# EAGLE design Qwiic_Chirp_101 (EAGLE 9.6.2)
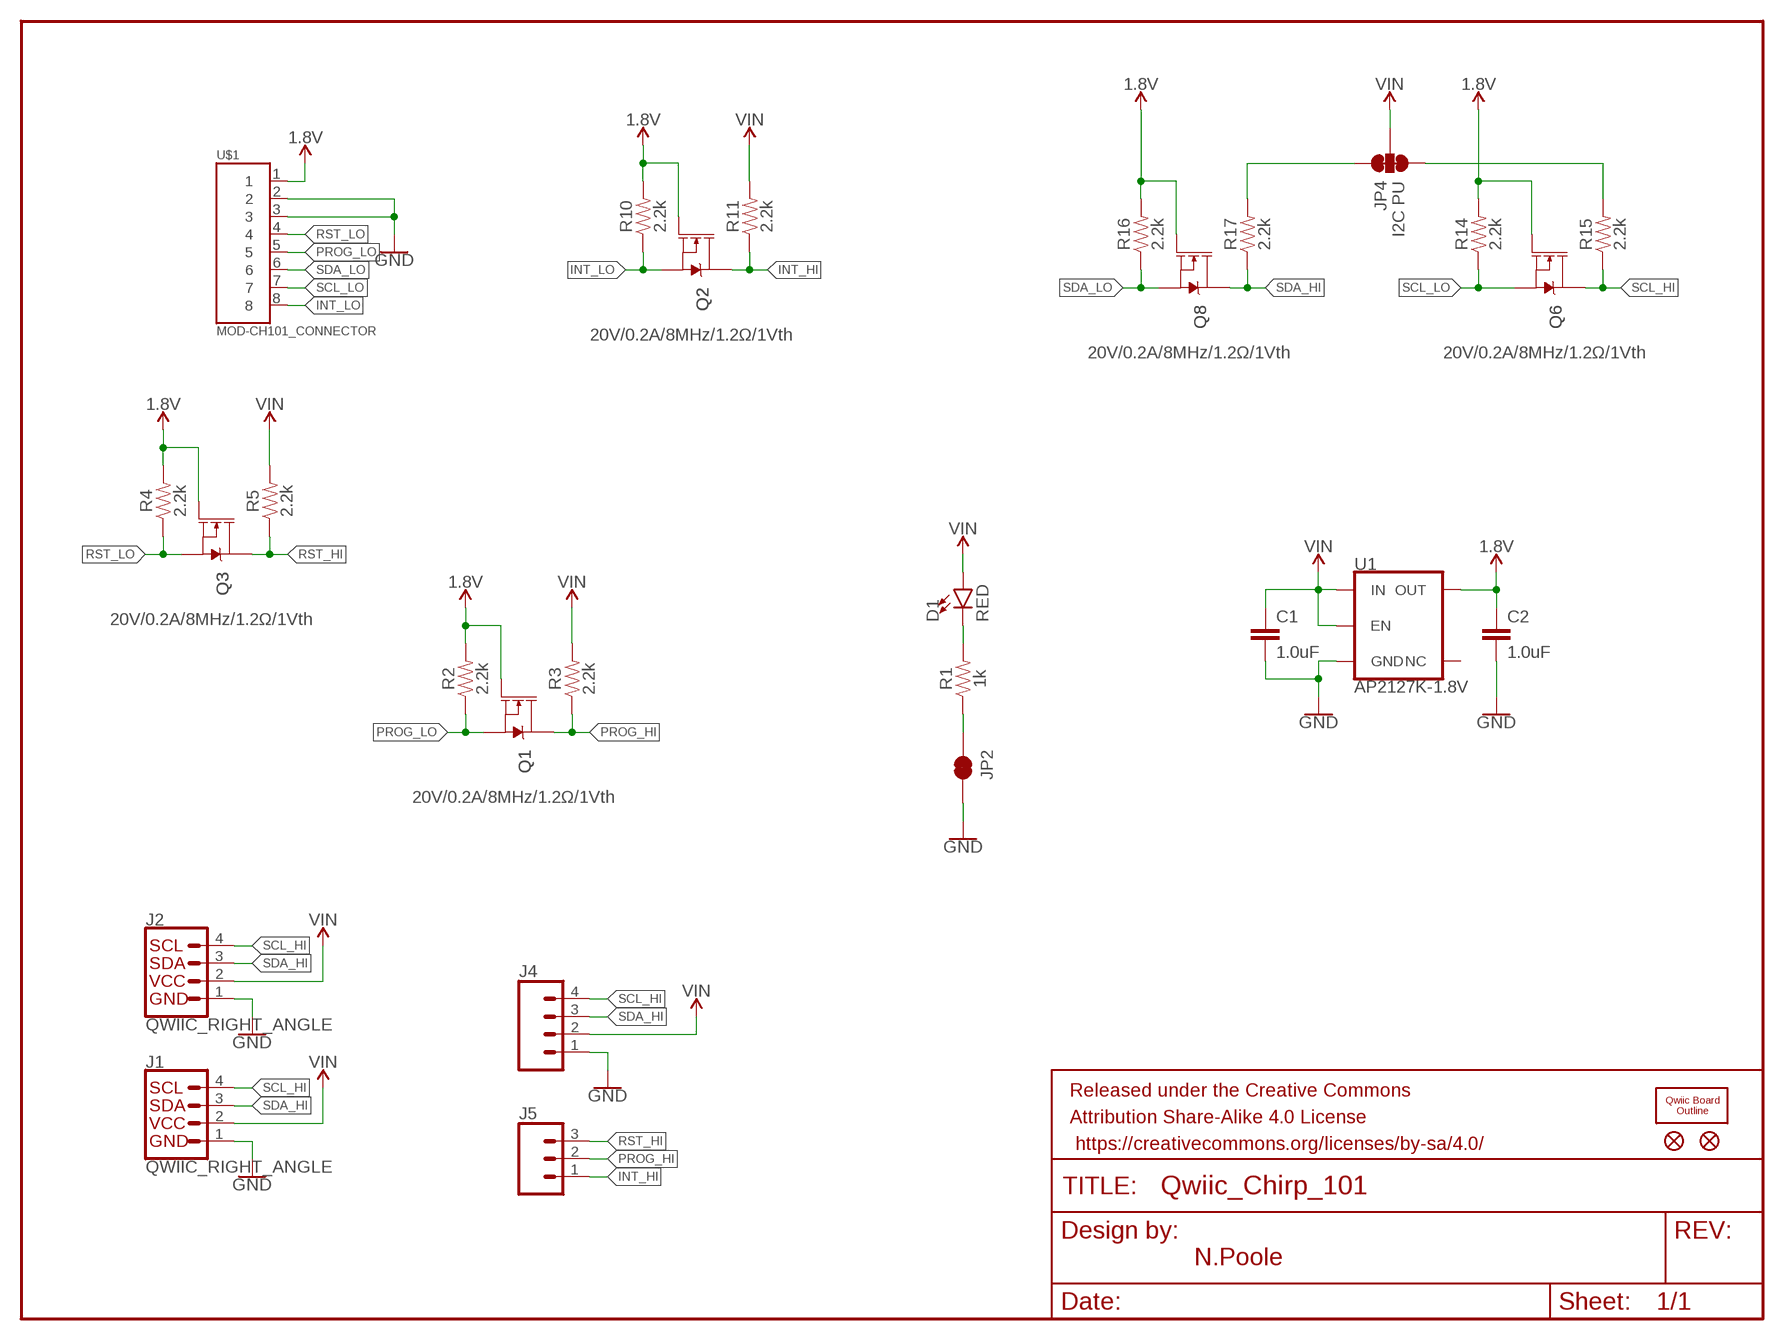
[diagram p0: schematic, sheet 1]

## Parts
C1  1.0uF  1.0UF-0603-16V-10%  [0603]
C2  1.0uF  1.0UF-0603-16V-10%  [0603]
D1  RED  LED-RED0603  [LED-0603]
FD1  FIDUCIALUFIDUCIAL  [FIDUCIAL-MICRO]
FD2  FIDUCIALUFIDUCIAL  [FIDUCIAL-MICRO]
FRAME1  FRAME-LETTERNO_PACKAGE  [DUMMY]
J1  QWIIC_RIGHT_ANGLE  QWIIC_CONNECTORJS-1MM  [JST04_1MM_RA]
J2  QWIIC_RIGHT_ANGLE  QWIIC_CONNECTORJS-1MM  [JST04_1MM_RA]
J4  CONN_041X04_NO_SILK  [1X04_NO_SILK]
J5  CONN_031X03_NO_SILK  [1X03_NO_SILK]
JP2  JUMPER-SMT_2_NC_TRACE_SILK  [SMT-JUMPER_2_NC_TRACE_SILK]
JP4  I2C PU  JUMPER-SMT_3_2-NC_TRACE_SILK  [SMT-JUMPER_3_2-NC_TRACE_SILK]
Q1  20V/0.2A/8MHz/1.2Ω/1Vth  MOSFET-NCH-RE1C002UN  [SOT-416FL]
Q2  20V/0.2A/8MHz/1.2Ω/1Vth  MOSFET-NCH-RE1C002UN  [SOT-416FL]
Q3  20V/0.2A/8MHz/1.2Ω/1Vth  MOSFET-NCH-RE1C002UN  [SOT-416FL]
Q6  20V/0.2A/8MHz/1.2Ω/1Vth  MOSFET-NCH-RE1C002UN  [SOT-416FL]
Q8  20V/0.2A/8MHz/1.2Ω/1Vth  MOSFET-NCH-RE1C002UN  [SOT-416FL]
R1  1k  1KOHM-0603-1/10W-1%  [0603]
R2  2.2k  2.2KOHM-0402T-1/16W-1%  [0402-TIGHT]
R3  2.2k  2.2KOHM-0402T-1/16W-1%  [0402-TIGHT]
R4  2.2k  2.2KOHM-0402T-1/16W-1%  [0402-TIGHT]
R5  2.2k  2.2KOHM-0402T-1/16W-1%  [0402-TIGHT]
R10  2.2k  2.2KOHM-0402T-1/16W-1%  [0402-TIGHT]
R11  2.2k  2.2KOHM-0402T-1/16W-1%  [0402-TIGHT]
R14  2.2k  2.2KOHM-0402T-1/16W-1%  [0402-TIGHT]
R15  2.2k  2.2KOHM-0402T-1/16W-1%  [0402-TIGHT]
R16  2.2k  2.2KOHM-0402T-1/16W-1%  [0402-TIGHT]
R17  2.2k  2.2KOHM-0402T-1/16W-1%  [0402-TIGHT]
U1  AP2127K-1.8V  V_REG_AP2127K-1.8V  [SOT23-5]
U$1  MOD-CH101_CONNECTOR  [FPC_MOLEX5034800800]
U$2  QWIIC_BOARD_OUTLINEH  [QWIIC_BOARD_MOUNT_HOLES]

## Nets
1.8V: C2.1 Q1.1(G) Q2.1(G) Q3.1(G) Q6.1(G) Q8.1(G) R2.2 R4.2 R10.2 R14.2 R16.2 U1.5(OUT) U$1.1
GND: C1.2 C2.2 J1.1 J2.1 J4.1 JP2.2 U1.2(GND) U$1.2 U$1.3
INT_HI: J5.1 Q2.3(D) R11.1
INT_LO: Q2.2(S) R10.1 U$1.8
N$1: D1.C R1.2
N$2: JP4.3 R15.2
N$3: JP4.1 R17.2
N$4: JP2.1 R1.1
PROG_HI: J5.2 Q1.3(D) R3.1
PROG_LO: Q1.2(S) R2.1 U$1.5
RST_HI: J5.3 Q3.3(D) R5.1
RST_LO: Q3.2(S) R4.1 U$1.4
SCL_HI: J1.4 J2.4 J4.4 Q6.3(D) R15.1
SCL_LO: Q6.2(S) R14.1 U$1.7
SDA_HI: J1.3 J2.3 J4.3 Q8.3(D) R17.1
SDA_LO: Q8.2(S) R16.1 U$1.6
VIN: C1.1 D1.A J1.2 J2.2 J4.2 JP4.2 R3.2 R5.2 R11.2 U1.1(IN) U1.3(EN)
Unconnected: U1.4(NC)

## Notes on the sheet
- N.Poole

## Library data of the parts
C1 C2 = SparkFun-Capacitors:1.0UF: 1µF ceramic capacitors; PROD_ID: CAP-00868
D1 = SparkFun-LED:LED-RED: Red SMD LED; PROD_ID: DIO-00819
FD1 FD2 = SparkFun-Aesthetics:FIDUCIAL: Fiducial Alignment Points
FRAME1 = SparkFun-Aesthetics:FRAME-LETTER: Schematic Frame - Letter; DESIGNER: Nobody; VERSION: v01
J1 J2 = SparkFun-Connectors:QWIIC_CONNECTOR: SparkFun I2C Standard Qwiic Connector An SMD 1mm pitch JST connector makes it easy and quick (get it? Qwiic?) to connect I2C devices to each other. The Qwiic system enables fast and solderless connection between popular platforms and various sensors and actuators. We carry 200mm, 100mm, 50mm, and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; PROD_ID: CONN-13694
J4 = SparkFun-Connectors:CONN_04: Multi connection point. Often used as Generic Header-pin footprint for 0.1 inch spaced/style header connections On any of the 0.1 inch spaced packages, you can populate with these: Break Away Headers - Straight (PRT-00116) Break Away Male Headers - Right Angle (PRT-00553) Female Headers (PRT-00115)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; PROD_ID: CONN-09696
J5 = SparkFun-Connectors:CONN_03: Multi connection point. Often used as Generic Header-pin footprint for 0.1 inch spaced/style header connections On any of the 0.1 inch spaced packages, you can populate with these: Break Away Headers - Straight (PRT-00116) Break Away Male Headers - Right Angle (PRT-00553) Female Headers (PRT-00115)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
JP2 = SparkFun-Jumpers:JUMPER-SMT_2_NC_TRACE: Normally closed trace jumper
JP4 = SparkFun-Jumpers:JUMPER-SMT_3_2-NC_TRACE: Normally closed trace jumper (2 of 2 connections) This jumper has a trace between all three pads so they are normally closed (NC). Use a razor knife to open the connection(s). For best results follow the IPC guidelines for cutting traces: Cutout at least 0.063 mm (0.005 in). Remove all loose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
Q1-Q3 Q6 Q8 = SparkFun-DiscreteSemi:MOSFET-NCH: N-channel MOSFETs Voltage controlled devices that allow control of high current outputs. SparkFun Products: SparkFun OpenScale SparkFun Digital Sandbox SparkFun Monster Moto Shield SparkFun MOSFET Power Controller; PROD_ID: TRANS_14399
R1 = SparkFun-Resistors:1KOHM: 1kΩ resistor; PROD_ID: RES-07856
R2-R5 R10 R11 R14-R17 = SparkFun-Resistors:2.2KOHM: 2.2kΩ resistor; PROD_ID: RES-14341
U1 = SparkFun-IC-Power:V_REG_AP2127: AP2127 - 300mA CMOS LDO Regulator w/ Enable The AP2127 is CMOS process low dropout linear regulator with enable function, the regulator delivers a guaranteed 300mA (min.) continuous load current. Features Output Voltage Accuracy: ±1.5% Output Current: 300mA (Min.) Foldback Short Current Protection: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; PROD_ID: VREG-14239
U$1 = SparkFun-Connectors:MOD-CH101_CONNECTOR
U$2 = SparkFun-Boards:QWIIC_BOARD_OUTLINE: Standard Outline of a Qwiic Board. Good for defining a spot on shields and board areas in which to mount a Qwiic Board.

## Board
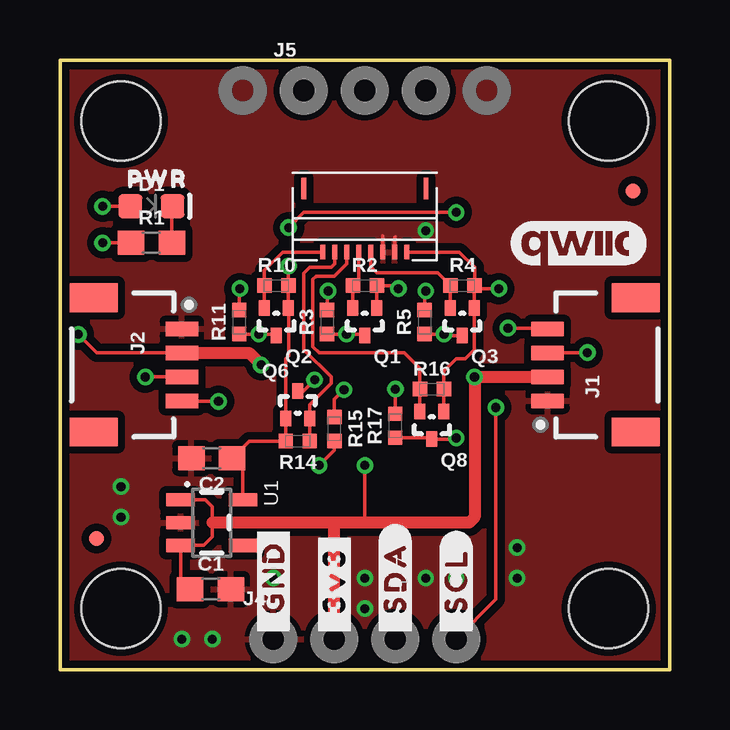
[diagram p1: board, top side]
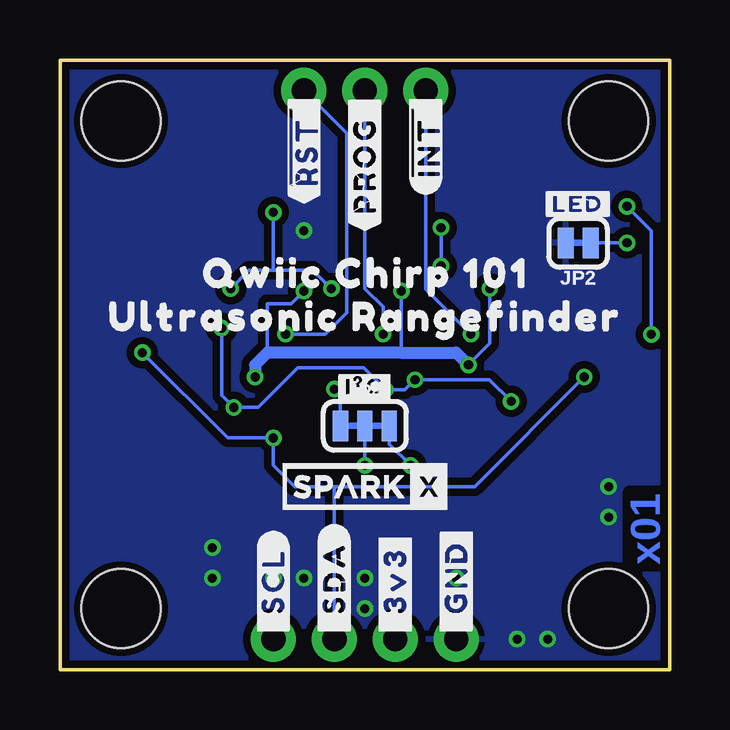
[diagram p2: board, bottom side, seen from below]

Size 25.4 x 25.4 mm. Coordinates in mm from the lower left corner, seen from the top.
Outline: 0,0 25.4,0 25.4,25.4 0,25.4 0,0
Copper layers (1*16): Top 0.035mm / dielectric 1.5mm / Bottom 0.035mm
Design rules "SparkFun-2-layer-PCBWay-LIMIT": minimum track width 6mil, minimum drill 0.3mm, track to track 6mil, track to pad 6mil, pad to pad 6mil, via to via 6mil, smd to smd 6mil, copper to edge 6mil, drill to drill 6mil, minimum pad ring 6mil, minimum via ring 6mil, stop-mask expansion 4mil, vias tented up to drill 25mil, thermal gap 10mil

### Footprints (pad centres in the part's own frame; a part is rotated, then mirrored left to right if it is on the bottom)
0603 = smd 1.1 x 1: 1 -0.85,0; 2 0.85,0
LED-0603 = smd 1 x 1: A -0.877,0; C 0.877,0
FIDUCIAL-MICRO = smd 0.635 x 0.635: 1 0,0
JST04_1MM_RA = smd 0.6 x 1.35: 1 -1.5,0; 2 -0.5,0; 3 0.5,0; 4 1.5,0 | smd 1.2 x 2: NC1 2.8,-3.675; NC2 -2.8,-3.675
1X04_NO_SILK = drill 1.016 pad 1.88: 1 0,0; 2 2.54,0; 3 5.08,0; 4 7.62,0
1X03_NO_SILK = drill 1.016 pad 1.88: 1 0,0; 2 2.54,0; 3 5.08,0
SMT-JUMPER_2_NC_TRACE_SILK = smd 0.66 x 1.27: 1 -0.521,0; 2 0.521,0
SMT-JUMPER_3_2-NC_TRACE_SILK = smd 0.635 x 1.27: 1 -1.016,0; 2 0,0; 3 1.016,0
SOT-416FL = smd 0.46 x 0.65: 1 -0.5,-1.1; 2 0.5,-1.1; 3 0,0.05
0402-TIGHT = smd 0.6 x 0.6: 1 -0.5,0; 2 0.5,0
SOT23-5 = smd 0.55 x 1.2: 1 -0.95,-1.3; 2 0,-1.3; 3 0.95,-1.3; 4 0.95,1.3; 5 -0.95,1.3
FPC_MOLEX5034800800 = smd 0.2 x 0.6: 1 -1.75,1.65; 2 -1.25,1.65; 3 -0.75,1.65; 4 -0.25,1.65; 5 0.25,1.65; 6 0.75,1.65; 7 1.25,1.65; 8 1.75,1.65 | smd 0.2 x 0.9: MNT1 -2.55,-1; MNT2 2.55,-1
QWIIC_BOARD_MOUNT_HOLES = hole 3.302: -10.16,10.16; 10.16,10.16; 10.16,-10.16; -10.16,-10.16

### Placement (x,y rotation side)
C1  6.27,3.35 0 top
C2  6.32,8.81 180 top
D1  3.81,19.3 0 top
FD1  1.52,5.46 0 top
FD2  23.88,19.94 0 top
FRAME1  0,0 0 top
J1  20.32,12.7 90 top
J2  5.08,12.7 270 top
J4  8.89,1.27 0 top
J5  10.16,24.13 0 top
JP2  3.81,17.78 180 bottom
JP4  12.7,10.16 0 bottom
Q1  12.7,13.97 180 top
Q2  9.02,13.97 180 top
Q3  16.76,13.97 180 top
Q6  9.91,11.56 0 top
Q8  15.49,9.65 180 top
R1  3.81,17.78 0 top
R2  12.7,16 0 top
R3  11.13,14.48 90 top
R4  16.76,16 0 top
R5  15.19,14.48 90 top
R10  9.02,16 0 top
R11  7.47,14.48 90 top
R14  9.91,9.53 180 top
R15  11.43,10.03 270 top
R16  15.49,11.68 0 top
R17  13.97,10.16 90 top
U1  6.32,6.12 270 top
U$1  12.7,19.05 180 top
U$2  12.7,12.7 0 top
U$3  [#_3V3#1]  11.43,1.27 90 top
U$4  [#_GND#0]  8.89,1.27 90 top
U$5  [#_SDA#2]  13.97,1.27 90 top
U$6  [#_SCL#3]  16.51,1.27 90 top
U$7  [QWIIC_CHIRP_1017]  20.32,16.51 0 bottom
U$8  [ULTRASONIC_RANGEFINDER8]  24.26,14.71 0 bottom
U$9  [#I�C#1019]  14.05,11.79 0 bottom
U$10  [#LED#1018]  5.41,19.41 0 bottom
U$11  [#_SCL#3]  16.51,1.27 90 bottom
U$12  [#_SDA#2]  13.97,1.27 90 bottom
U$13  [#_3V3#1]  11.43,1.27 90 bottom
U$14  [#_GND#0]  8.89,1.27 90 bottom
U$15  [##INT_##0]  10.16,19.81 90 bottom
U$16  [##RST_##1]  15.24,19.43 90 bottom
U$17  [#PROG_#5]  12.7,18.29 90 bottom
U$18  [SPARKX-SMALL]  12.7,7.62 0 bottom
U$19  [QWIIC_COPYRIGHT_SMALL]  21.59,17.78 0 top
U$20  [PWR0]  2.29,20.45 0 top

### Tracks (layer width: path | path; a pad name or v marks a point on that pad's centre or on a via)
1.8V  (via drill 0.38)
  Top 0.152: Q8.1 R16.2 15.99,12.44 16.51,12.95 16.89,12.95 17.26,13.33 Q3.1 R4.2 | Q1.1 R2.2 13.97,16 v14.1,15.88 | U$1.1 16.64,17.4 17.27,16.76 17.27,16.01 R4.2 | v18.29,15.88 17.39,15.88 R4.2 | v9.53,16.82 9.52,16.81 R10.2 Q2.1 9.53,13.08 9.41,12.96 Q6.1 R14.2 7.89,9.53 C2.1 7.62,8.36 U1.5 | v16.51,19.05 10.16,19.05 v9.53,18.41
  Bottom 0.152: 16.51,16.64 17.53,16.64 v18.29,15.88 | 16.51,16.64 14.86,16.64 v14.1,15.88 | v9.53,16.82 v9.53,18.41 | v16.51,19.05 16.51,16.64
GND  (via drill 0.38)
  Top 0.152: U$1.2 13.95,18.01 13.97,18.03 | U$1.3 13.45,18.07
  other vias: 15.24,18.29 12.7,3.81 12.7,2.54 19.05,5.08 19.05,3.81 15.24,3.81 16.51,3.81 2.54,7.62 2.54,6.35 5.08,1.27 6.35,1.27 8.89,3.81
  pour Top (isolate 0.305): 0,25.4 25.4,25.4 25.4,0 0,0
  pour Bottom (isolate 0.305): 0,25.4 25.4,25.4 25.4,0 0,0
INT_HI  (via drill 0.38)
  Top 0.152: Q2.3 8.96,13.98 v8.28,13.98 R11.1
  Bottom 0.152: v8.28,13.98 10.16,15.86 J5.1
INT_LO
  Top 0.152: Q2.2 R10.1 8.52,16.64 9.27,17.4 U$1.8
N$1
  Top 0.152: R1.2 4.66,19.28 D1.C
N$2  (via drill 0.38)
  Top 0.152: R15.2 11.43,9.14 v10.79,8.51
  Bottom 0.152: v10.79,8.51 11.68,9.4 JP4.3
N$3  (via drill 0.38)
  Top 0.152: R17.2 v13.97,11.68
  Bottom 0.152: v13.97,11.68 13.72,11.43 JP4.1
N$4  (via drill 0.38)
  Top 0.152: R1.1 v1.78,17.78
  Bottom 0.152: v1.78,17.78 JP2.1
PROG_HI  (via drill 0.38)
  Top 0.152: Q1.3 12.64,13.98 v11.94,13.98 R3.1
  Bottom 0.152: v11.94,13.98 11.94,15.11 12.7,15.88 J5.2
PROG_LO
  Top 0.152: Q1.2 R2.1 12.45,16.25 U$1.5
RST_HI  (via drill 0.38)
  Top 0.152: R5.1 v16,13.98 16.06,13.92 Q3.3
  Bottom 0.152: J5.3 13.46,22.35 13.46,14.86 14.34,13.98 v16,13.98
RST_LO
  Top 0.152: Q3.2 R4.1 15.73,16.53 13.21,16.53 12.95,16.79 U$1.4
SCL_HI  (via drill 0.38)
  Top 0.152: Q6.3 10.14,11.61 v10.61,12.08 | v6.6,11.18 5.1,11.18 J2.4 | R15.1 11.43,11.26 v11.83,11.66 | v18.67,14.22 20.3,14.22 J1.4 | v18.16,10.92 18.16,2.92 J4.4
  Bottom 0.152: v6.6,11.18 7.51,12.08 v10.61,12.08 11.03,11.66 v11.83,11.66 12.75,12.57 15.49,12.57 17.14,10.92 v18.16,10.92 18.67,11.43 v18.67,14.22
SCL_LO
  Top 0.152: U$1.7 11.45,16.91 11.3,16.76 10.41,16.76 10.16,16.51 10.16,13.34 11.3,12.19 11.3,11.94 10.41,11.04 Q6.2 R14.1
SDA_HI  (via drill 0.38)
  Top 0.152: R17.1 15.44,9.66 Q8.3 16.46,9.6 v16.51,9.65 | v21.97,13.21 v21.96,13.2 J1.3 | J2.3 v3.56,12.2 v3.56,12.19
  Bottom 0.152: v21.97,13.21 18.41,9.65 v16.51,9.65 16.51,8.51 15.62,7.62 13.97,7.62 | v3.56,12.19 8.13,7.62 13.97,7.62 | J4.3 13.97,7.62
SDA_LO
  Top 0.152: Q8.2 R16.1 14.99,12.56 14.35,13.21 10.79,13.21 10.54,13.46 10.54,16.26 10.67,16.38 11.43,16.38 11.95,16.9 U$1.6
VIN  (via drill 0.38)
  Top 0.152: 11.75,1.59 J4.2 | R3.2 11.12,15.72 v11.18,15.77 | R11.2 7.47,15.85 v7.49,15.88 | R5.2 15.19,15.72 v15.24,15.77 | D1.A v1.78,19.3 | J2.2 1.53,13.2 v0.76,13.97 | U1.1 5.04,7.09 6.04,7.09 6.35,6.78 6.35,6.12 6.35,5.54 5.98,5.17 U1.3 5.02,3.75 C1.1 | v12.7,8.51 12.7,6.12
  Top 0.508: J2.2 7.88,13.2 v8.38,12.7 | J1.2 v17.27,12.19 17.27,6.35 17.04,6.12 12.7,6.12 11.43,6.12 | 11.43,6.12 6.35,6.12 | J4.2 11.43,6.12
  Bottom 0.152: v7.49,15.88 7.49,13.59 v8.38,12.7 | v15.24,15.77 15.77,15.24 16.76,15.24 16.76,13.21 | 11.18,13.21 v11.18,15.77 | v0.76,13.97 0.76,18.29 v1.78,19.3 | JP4.2 v12.7,8.51
  Bottom 0.508: v8.38,12.7 8.89,13.21 11.18,13.21 16.76,13.21 17.27,12.7 v17.27,12.19

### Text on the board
Bottom: x01

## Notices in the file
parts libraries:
SparkFun-Aesthetics: Licensing: Creative Commons ShareAlike 4.0 International - https://creativecommons.org/licenses/by-sa/4.0
SparkFun-Aesthetics: Released under the Creative Commons Attribution Share-Alike 4.0 License
SparkFun-Aesthetics: https://creativecommons.org/licenses/by-sa/4.0
